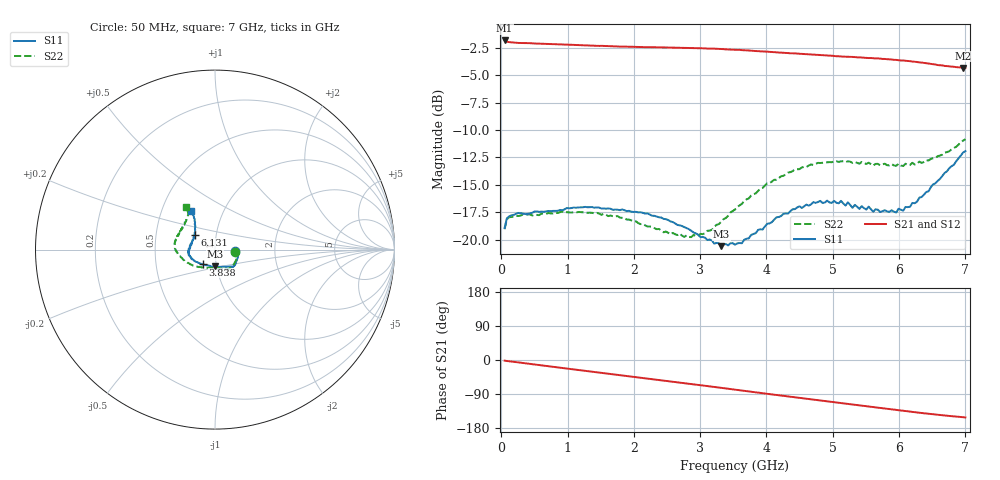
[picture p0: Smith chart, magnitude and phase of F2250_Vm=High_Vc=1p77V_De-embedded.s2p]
! Integrated Device Technology
! Corporate Headquarters
! 6024 Silver Creek Valley Road
! San Jose, CA 95138  USA
! Phone:  1-408-284-8200
! Toll Free:  1-800-223-1366
! Webpage:  http://www.idt.com/
! Timing and RF Division
! 515 Groton Road, Suite 102
! Westford, MA 01886-6024
! Device:  F2250
! Description: Voltage Variable RF Attenuator
! Frequency:  50.0 -  6000.00 MHz
! Package:  3x3 mm Thin QFN Plastic Package: 16 pin
! Ports:  2 RF, 3 DC
!  Pin  1  = GND
!  Pin  2  = NC
!  Pin  3  = RF1  = Port 1
!  Pin  4  = NC
!  Pin  5  = GND
!  Pin  6  = GND
!  Pin  7  = GND
!  Pin  8  = GND
!  Pin  9  = NC
!  Pin 10  = RF2  = Port 2
!  Pin 11  = NC
!  Pin 12  = GND
!  Pin 13  = GND
!  Pin 14  = VCNTRL
!  Pin 15  = VDD
!  Pin 16  = VMODE
! Vcntrl:  1.770 Volts
! Vmode:  +3.300 Volts
! Vdd:  +3.30  Volts
! Current:  1.326 mA
! Data:  The device was measured on a the F2250 evaluation board which has
!  individual transmission lines to the RF pins.  Data was collected
!  using a calibrated network analyzer.  The evaluation board was
!  de-embedded using a TRL calibration technique.
!  The reference plane is the edge of the package pin.
! Misc:  SN 10
!  Action Tracker AT0258
! Date Measured:  2014-11-26
! Date:  2015-10-15  MJV
! Note:
!  Integrated Device Technology supplies this data as a sample of measured
!  data at the package pin for this product.  Your particular data for this
!  product may vary.
!  Data was taken at 25 degrees C.
!  Integrated Device Technology reserves the right to change this data at anytime.
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# GHz S dB R 50
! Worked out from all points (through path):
!   201 points, 50 MHz to 7 GHz, reference 50 ohm
!   highest |S21| = -1.80 dB at 50 MHz (marker M1); lowest = -4.3 dB at 6.965 GHz (marker M2)
!   group delay of S21, straight-line fit = 60.9 ps
!   lowest |S11| = -20.6 dB at 3.317 GHz (marker M3), VSWR 1.21, Z = 49.2 - j9.25 ohm
!   |S11| at or under -10 dB: start of sweep to end of sweep
!   |S22| runs from -19.8 to -10.8 dB; largest |S21 - S12| = 0.0019
!   S11 on the Smith chart (normalised r, x): 50 MHz: 1.25, -0.02; 3.838 GHz: 0.86, -0.14; 6.131 GHz: 0.79, +0.13; 7 GHz: 0.70, +0.33
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0.05  -18.93 -4.6  -1.80 -1.9  -1.80 -1.9  -19.06 -6.0
0.08475  -18.06 -4.6  -1.92 -2.6  -1.93 -2.5  -18.14 -5.6
0.2585  -17.57 -10.4  -2.03 -6.4  -2.02 -6.4  -17.85 -13.0
1.2315  -17.05 -38.1  -2.23 -27.9  -2.23 -27.9  -17.51 -49.2
1.75275  -17.28 -44.9  -2.36 -39.0  -2.35 -39.0  -17.85 -60.6
2.37825  -17.97 -48.7  -2.43 -52.5  -2.44 -52.5  -19.03 -72.9
2.86475  -19.20 -60.1  -2.50 -63.3  -2.50 -63.3  -19.78 -94.8
3.1775  -20.10 -77.3  -2.55 -70.3  -2.55 -70.4  -19.11 -115.4
3.3165  -20.61 -89.6  -2.58 -73.5  -2.59 -73.6  -18.38 -124.5
3.525  -20.48 -106.1  -2.66 -78.2  -2.66 -78.3  -17.26 -136.3
3.83775  -19.42 -129.4  -2.77 -85.3  -2.77 -85.3  -15.79 -151.3
4.1505  -17.97 -146.9  -2.90 -92.3  -2.89 -92.3  -14.53 -164.3
4.32425  -17.63 -153.5  -2.96 -96.1  -2.97 -96.1  -13.88 -170.0
4.7065  -16.59 -166.8  -3.10 -104.5  -3.10 -104.5  -13.18 -180.0
5.1235  -16.47 -177.4  -3.27 -113.6  -3.27 -113.7  -12.85 170.0
5.29725  -17.10 177.0  -3.31 -117.4  -3.31 -117.4  -13.00 166.5
5.332  -16.84 175.6  -3.33 -118.2  -3.33 -118.2  -12.91 165.6
5.85325  -17.47 156.9  -3.53 -129.4  -3.53 -129.5  -13.22 151.7
6.13125  -17.04 143.9  -3.68 -135.4  -3.69 -135.5  -13.20 144.1
6.54825  -14.86 128.8  -4.00 -144.0  -4.01 -144.2  -12.54 130.5
6.96525  -12.05 121.7  -4.31 -151.0  -4.32 -151.1  -10.96 124.6
7  -11.92 121.3  -4.31 -151.5  -4.33 -151.6  -10.84 123.8
